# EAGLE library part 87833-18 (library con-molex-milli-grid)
HEADER
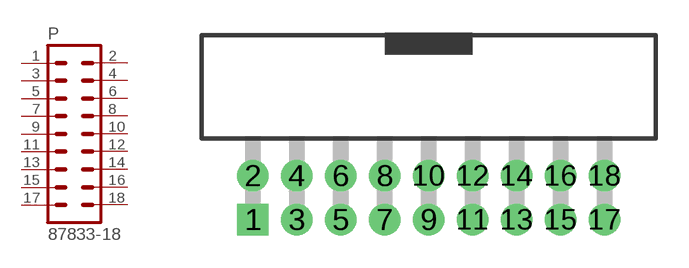
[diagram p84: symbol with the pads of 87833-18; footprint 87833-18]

Designator prefix P

## 87833-18  [87833-18]
1  1  pas
2  2  pas
3  3  pas
4  4  pas
5  5  pas
6  6  pas
7  7  pas
8  8  pas
9  9  pas
10  10  pas
11  11  pas
12  12  pas
13  13  pas
14  14  pas
15  15  pas
16  16  pas
17  17  pas
18  18  pas

## Footprint 87833-18 (pad centres in mm)
HEADER Dual Row, Shrouded, Right Angle
drill 0.914 square: 1 -8,-1
drill 0.914: 2 -8,1; 3 -6,-1; 4 -6,1; 5 -4,-1; 6 -4,1; 7 -2,-1; 8 -2,1; 9 0,-1; 10 0,1; 11 2,-1; 12 2,1; 13 4,-1; 14 4,1; 15 6,-1; 16 6,1; 17 8,-1; 18 8,1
